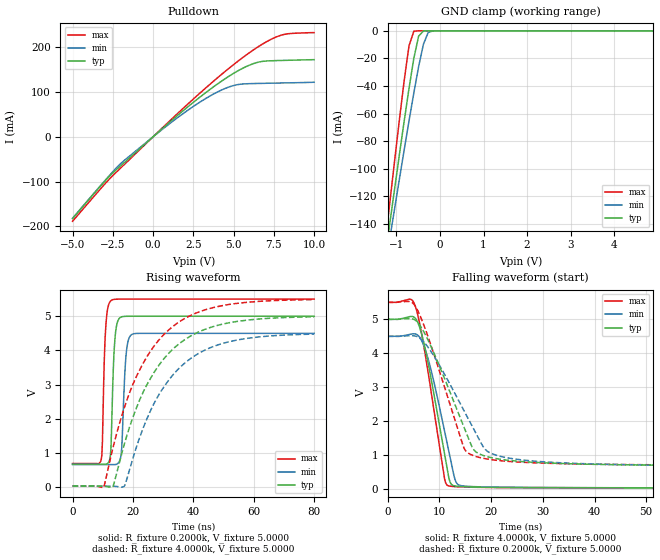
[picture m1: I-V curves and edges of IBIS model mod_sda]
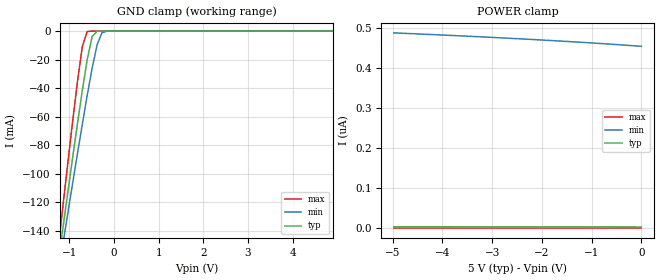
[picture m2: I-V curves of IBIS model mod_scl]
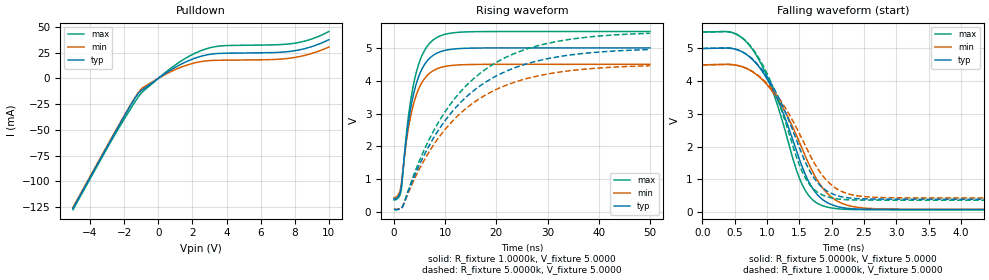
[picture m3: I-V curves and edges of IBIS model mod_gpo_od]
| IBIS (I/O, Buffer, Information, Specification) Model, officially
| electronic behavioral standard for Buffer structures of digital pins.
[IBIS ver]  4.0
[File name] st25dv04kc_so8_5v0.ibs
[File Rev]  1.0
[Date]   20 March 2024
[Notes]
   (Note1)  This IBIS model includes the SO8 package data
   (Note2)  This IBIS model has some Notes about the non-monotonicity
   of the I-V curves, but they are not indicative of problems
   inside the model;
[Disclaimer]
   Customers are solely responsible for all aspects of their
   own product designs or applications using this IBIS Model.
   STMicroelectronics assumes no liability for Custmer Designs
   and applications associated to this IBIS Model.
   In the use of this IBIS Model Customer shall not modify,
   disassemble, alter this Model in whole or in part.
   If Customers do not accept these terms, the IBIS Model
   may not be used. For any problems or modifications please
   contact STMicroelectronics (www.st.com).
[Copyright] (c) 2024 STMicroelectronics
|   Component ST25DV04K
[Component] ST25DV04K
[Manufacturer] STMicroelectronics
[Package]
| variable  typ   min   max
R_pkg   0.0   0.0   0.0
L_pkg   0.0H   0.0H   0.0H
C_pkg   0.0F   0.0F   0.0F
[Pin]  signal_name  model_name   R_pin   L_pin   C_pin
1   VEH   NC   0.0   0.0   0.0
2   AC0   NC   0.0   0.0   0.0
3   AC1   NC   0.0   0.0   0.0
4   VSS   GND   130.95m   2.182nH   0.287pF
5   SDA   mod_sda   130.79m   2.182nH   0.286pF
6   SCL   mod_scl   85.32m   1.589nH   0.354pF
7   GPO   mod_gpo_od   84.54m   1.583nH   0.355pF
8   VCC   POWER   124.14m   2.142nH   0.284pF
| Models and submodels in the file (3): mod_sda (I/O_open_drain), mod_scl (Input), mod_gpo_od (Open_drain)
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|   Model mod_sda
[Model]   mod_sda
Model_type I/O_open_drain
Polarity   Non-Inverting
Enable   Active-Low
Vinl   =  1.250V
Vinh   =  3.750V
Vmeas   =  2.500V
Cref   =  30pF
Rref   =  4.0k
Vref   =  5.00V
C_comp   3.063pF   2.925pF   3.207pF
[Model Spec]
Vinl   1.250V   1.125V   1.375V
Vinh   3.750V   3.375V   4.125V
Vmeas   2.500V   2.250V   2.750V
[Temperature Range]  25.0000   85.0000   -40.0000
[Voltage Range]   5.0000V   4.5000V   5.5000V
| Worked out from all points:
|   slope of the pulldown table from 0 to 0.75 V, typ, clamps not added: 31.4 ohm
|   GND clamp passes 1 mA (typ) near -0.41 V on its own axis
|   rising waveform, R_fixture 0.2000k, V_fixture 5.0000: 20-80 % time 1.01ns typ, 1.16ns min, 933ps max; typ from 0.678 V to 5 V
|   rising waveform, R_fixture 4.0000k, V_fixture 5.0000: 20-80 % time 16.3ns typ, 16.4ns min, 16.2ns max; typ from 0.039 V to 4.98 V
|   falling waveform, R_fixture 4.0000k, V_fixture 5.0000: 20-80 % time 3.58ns typ, 3.85ns min, 3.38ns max; typ from 5 V to 0.039 V
|   falling waveform, R_fixture 0.2000k, V_fixture 5.0000: 20-80 % time 6.92ns typ, 8.08ns min, 6.1ns max; typ from 5 V to 0.687 V
[Pulldown]
|Voltage   I(typ)   I(min)   I(max)
-5V       -182.8mA   -182mA     -188.6mA
-2.92V    -96.28mA   -94.96mA   -102.4mA
-1.96V    -63.18mA   -58.09mA   -67.85mA
1.4V      44.05mA    39.47mA    47.88mA
2.68V     82.06mA    72.08mA    90.15mA
3.64V     108.6mA    93.23mA    120.6mA
4.76V     136.3mA    111.8mA    154.3mA
5.72V     155.8mA    118.2mA    180.9mA
6.52V     166.5mA    119.1mA    200.9mA
7.32V     169.7mA    119.7mA    217.5mA
8.28V     170.7mA    120.4mA    229.5mA
10V       172.2mA    121.8mA    232.7mA
[GND_clamp]
|Voltage   I(typ)   I(min)   I(max)
-5V       -1.048A    -930.3mA   -1.231A
-1.26V    -164.5mA   -172mA     -154.8mA
-1.15V    -139.2mA   -150.2mA   -124.1mA
-1.04V    -114.2mA   -128.6mA   -93.8mA
-820mV    -65.05mA   -85.99mA   -35.6mA
-710mV    -41.55mA   -65.17mA   -10.77mA
-600mV    -19.87mA   -44.97mA   -297.8uA
-490mV    -3.87mA    -25.93mA   -1.514uA
-380mV    -108.6uA   -9.705mA   -7.328nA
-270mV    -1.71uA    -1.125mA   -37.78pA
-160mV    -27.95nA   -41.15uA   -2.358pA
4.9V      2.999nA    458.7nA    13.02pA
[Ramp]
| variable   typ   min   max
dV/dt_r   1.8264/1.0721n   1.5694/1.2261n   2.0761/0.6678n
dV/dt_f   1.8129/12.2723n   1.5491/15.6301n   2.0669/10.4029n
R_load = 50.0000
[Rising Waveform]
R_fixture= 0.2000k
V_fixture= 5.0000
V_fixture_min= 4.5000
V_fixture_max= 5.5000
|time   V(typ)   V(min)   V(max)
0s        678.1mV    665.8mV    696.8mV
9.5ns     678.1mV    665.8mV    813.8mV
11.1ns    677.1mV    665.8mV    4.812V
12.9ns    1.616V     665.8mV    5.467V
13.7ns    3.869V     664.5mV    5.491V
14.5ns    4.685V     672.5mV    5.498V
16.1ns    4.977V     955.7mV    5.5V
17.7ns    4.998V     3.842V     5.5V
19.5ns    5V         4.459V     5.5V
80ns      5V         4.5V       5.5V
[Rising Waveform]
R_fixture= 4.0000k
V_fixture= 5.0000
V_fixture_min= 4.5000
V_fixture_max= 5.5000
|time   V(typ)   V(min)   V(max)
0s        38.54mV    38.14mV    39.35mV
10.2ns    38.33mV    38.14mV    -14.54mV
13.3ns    8.988mV    37.63mV    1.124V
17.1ns    1.248V     28.99mV    2.315V
21.1ns    2.31V      1.162V     3.23V
25.1ns    3.074V     2.101V     3.884V
33.5ns    4.061V     3.312V     4.721V
40.7ns    4.497V     3.859V     5.086V
49.9ns    4.774V     4.21V      5.315V
80ns      4.984V     4.479V     5.487V
[Falling Waveform]
R_fixture= 4.0000k
V_fixture= 5.0000
V_fixture_min= 4.5000
V_fixture_max= 5.5000
|time   V(typ)   V(min)   V(max)
0s        5V         4.5V       5.5V
4.3ns     5.081V     4.56V      5.596V
5.4ns     5.02V      4.569V     5.36V
7.8ns     3.727V     3.847V     3.459V
11ns      1.032V     1.709V     304mV
11.6ns    515.6mV    1.272V     107.3mV
12.2ns    165.7mV    838.6mV    85.48mV
13.2ns    91.11mV    213.9mV    72.84mV
14.6ns    74.58mV    95.28mV    63.49mV
80ns      39.17mV    39.03mV    39.81mV
[Falling Waveform]
R_fixture= 0.2000k
V_fixture= 5.0000
V_fixture_min= 4.5000
V_fixture_max= 5.5000
|time   V(typ)   V(min)   V(max)
0s        5V         4.5V       5.5V
4.2ns     5.023V     4.52V      5.524V
5.5ns     4.956V     4.502V     5.348V
6.9ns     4.658V     4.35V      4.867V
8.7ns     4.09V      3.979V     4.088V
14.7ns    1.845V     2.325V     1.236V
16.5ns    1.194V     1.803V     992mV
19.3ns    954.7mV    1.114V     886.2mV
25.7ns    816.4mV    866mV      794.7mV
80ns      687.1mV    678.8mV    703.2mV
|   Model mod_scl
[Model]   mod_scl
Model_type Input
Vinl   =   1.250V
Vinh   =   3.750V
C_comp   2.118pF   2.024pF   2.219pF
[Model Spec]
Vinl   1.250V   1.125V   1.375V
Vinh   3.750V   3.375V   4.125V
[Temperature Range]  25.0000   85.0000   -40.0000
[Voltage Range]   5.0000V   4.5000V   5.5000V
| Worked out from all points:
|   GND clamp passes 1 mA (typ) near -0.41 V on its own axis
[GND_clamp]
|Voltage   I(typ)   I(min)   I(max)
-5V       -1.048A    -930.3mA   -1.231A
-1.26V    -164.5mA   -172mA     -154.8mA
-1.15V    -139.2mA   -150.2mA   -124.1mA
-1.04V    -114.2mA   -128.6mA   -93.8mA
-820mV    -65.05mA   -85.99mA   -35.6mA
-710mV    -41.55mA   -65.17mA   -10.77mA
-600mV    -19.87mA   -44.97mA   -297.8uA
-490mV    -3.87mA    -25.93mA   -1.514uA
-380mV    -108.6uA   -9.705mA   -7.328nA
-270mV    -1.71uA    -1.125mA   -37.78pA
-160mV    -27.95nA   -41.15uA   -2.358pA
4.9V      2.999nA    458.7nA    13.02pA
[POWER_clamp]
|Voltage   I(typ)   I(min)   I(max)
-4.98V    3.496nA    488.8nA    24.75pA
-4.02V    3.419nA    483.6nA    22.75pA
-3.3V     3.357nA    479.4nA    21.25pA
-2.16V    3.251nA    472.1nA    18.86pA
-1.44V    3.177nA    467nA      17.35pA
-840mV    3.112nA    462.4nA    16.08pA
-240mV    3.041nA    457.4nA    14.81pA
0V        3.011nA    455.2nA    14.3pA
|   Model mod_gpo_od
[Model]   mod_gpo_od
Model_type Open_drain
Polarity   Non-Inverting
Enable   Active-Low
Vmeas  =   2.500V
Cref   =   30.0pF
Rref   =   5.0k
Vref   =   5.00V
C_comp   2.219pF   2.119pF   2.324pF
[Model Spec]
Vmeas   2.500V   2.250V   2.750V
[Temperature Range]  25.0000   85.0000   -40.0000
[Voltage Range]   5.0000V   4.5000V   5.5000V
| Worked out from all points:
|   slope of the pulldown table from 0 to 0.75 V, typ, clamps not added: 90 ohm
|   rising waveform, R_fixture 1.0000k, V_fixture 5.0000: 20-80 % time 2.92ns typ, 2.93ns min, 2.92ns max; typ from 0.398 V to 5 V
|   rising waveform, R_fixture 5.0000k, V_fixture 5.0000: 20-80 % time 14.2ns typ, 14.2ns min, 14.2ns max; typ from 0.082 V to 4.95 V
|   falling waveform, R_fixture 5.0000k, V_fixture 5.0000: 20-80 % time 595ps typ, 670ps min, 540ps max; typ from 5 V to 0.082 V
|   falling waveform, R_fixture 1.0000k, V_fixture 5.0000: 20-80 % time 627ps typ, 703ps min, 570ps max; typ from 5 V to 0.398 V
[Pulldown]
|Voltage   I(typ)   I(min)   I(max)
-5V       -126.4mA   -125.4mA   -127.7mA
-2.76V    -59.4mA    -58.52mA   -60.95mA
-1.64V    -26.67mA   -26.1mA    -30.09mA
-1.16V    -14.37mA   -13.61mA   -17.7mA
-840mV    -9.978mA   -8.24mA    -11.83mA
1.24V     12.97mA    10.27mA    15.84mA
2.04V     18.98mA    14.66mA    23.56mA
2.84V     22.82mA    17.07mA    28.89mA
3.8V      24.42mA    17.71mA    31.75mA
7.96V     26.81mA    20.25mA    34.14mA
8.92V     30.49mA    23.86mA    37.91mA
10V       37.62mA    30.45mA    45.6mA
[Ramp]
| variable   typ   min   max
dV/dt_r   0.7324/1.0407n   0.5300/1.0367n   0.9553/1.0494n
dV/dt_f   0.7319/0.9340n   0.5302/0.9319n   0.9548/0.9587n
R_load = 50.0000
[Rising Waveform]
R_fixture= 1.0000k
V_fixture= 5.0000
V_fixture_min= 4.5000
V_fixture_max= 5.5000
|time   V(typ)   V(min)   V(max)
0s        398.4mV    437.1mV    368.6mV
900ps     485mV      540.4mV    438.9mV
1.4ns     734.3mV    819.6mV    652.3mV
2.8ns     2.713V     2.534V     2.885V
3.5ns     3.36V      3.091V     3.626V
4.3ns     3.88V      3.537V     4.221V
5.9ns     4.478V     4.05V      4.904V
8ns       4.808V     4.335V     5.281V
14.2ns    4.99V      4.491V     5.489V
50ns      5V         4.5V       5.5V
[Rising Waveform]
R_fixture= 5.0000k
V_fixture= 5.0000
V_fixture_min= 4.5000
V_fixture_max= 5.5000
|time   V(typ)   V(min)   V(max)
0s        82.48mV    90.91mV    76.04mV
1.7ns     168.6mV    178.4mV    157.6mV
5.5ns     1.61V      1.465V     1.755V
9.7ns     2.724V     2.462V     2.987V
13.7ns    3.445V     3.106V     3.783V
18.1ns    3.977V     3.583V     4.372V
23.35ns   4.38V      3.944V     4.816V
30.35ns   4.682V     4.215V     5.15V
38.15ns   4.849V     4.364V     5.334V
50ns      4.951V     4.456V     5.446V
[Falling Waveform]
R_fixture= 5.0000k
V_fixture= 5.0000
V_fixture_min= 4.5000
V_fixture_max= 5.5000
|time   V(typ)   V(min)   V(max)
0s        5V         4.5V       5.5V
480ps     4.994V     4.503V     5.475V
780ps     4.656V     4.285V     4.965V
1.14ns    3.546V     3.532V     3.408V
1.56ns    1.308V     1.863V     781.8mV
1.74ns    632.3mV    1.108V     324.4mV
1.98ns    247.6mV    491.9mV    137.6mV
2.31ns    107.7mV    181.2mV    82.45mV
2.88ns    83.42mV    97.32mV    76.16mV
15ns      82.48mV    90.9mV     76.04mV
[Falling Waveform]
R_fixture= 1.0000k
V_fixture= 5.0000
V_fixture_min= 4.5000
V_fixture_max= 5.5000
|time   V(typ)   V(min)   V(max)
0s        5V         4.5V       5.5V
465ps     4.998V     4.505V     5.483V
765ps     4.697V     4.311V     5.027V
1.155ns   3.605V     3.567V     3.504V
1.455ns   2.21V      2.584V     1.694V
1.605ns   1.482V     1.979V     1.008V
1.815ns   830.8mV    1.238V     569mV
2.055ns   525.6mV    744.7mV    417mV
2.955ns   399.1mV    442mV      368.7mV
15ns      398.4mV    437.1mV    368.6mV
